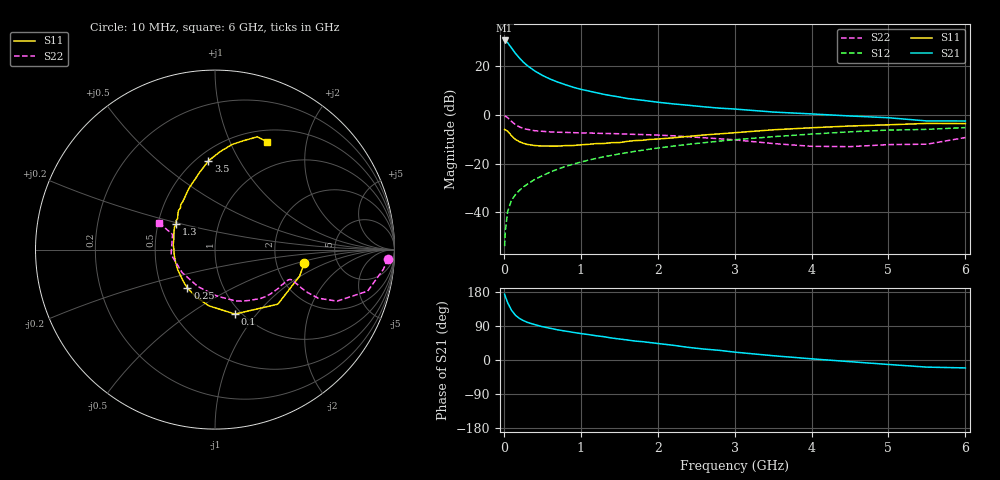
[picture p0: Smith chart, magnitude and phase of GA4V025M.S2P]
! Infineon Technologies  Discrete & RF Semiconductors
! BF775
! Si NPN RF Bipolar Junction Transistor in SOT23
! VCE = 4 V  IC = 25 mA
! Common Emitter S-Parameters:  May  1996
# GHz  S  MA  R  50
!  f  S11  S21  S12  S22
! GHz  MAG  ANG  MAG  ANG  MAG  ANG  MAG  ANG
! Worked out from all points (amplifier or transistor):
!   36 points, 10 MHz to 6 GHz, reference 50 ohm
!   highest |S21| = 30.7 dB at 10 MHz (marker M1)
!   |S21| within 3 dB of that: start of sweep to 97.65 MHz
!   unconditionally stable (mu >= 1): 338 MHz to 2.928 GHz
!   at 250 MHz: K = 0.92, MSG = 25.8 dB, |S12| = -29.7 dB
!   at 1.4 GHz: K = 1.12, MAG = 10.2 dB, |S12| = -16.6 dB
!   at 6 GHz: K = 0.94, MSG = 1.4 dB, |S12| = -5.2 dB
!   S11 on the Smith chart (normalised r, x): 10 MHz: 2.89, -0.59; 100 MHz: 0.93, -0.78; 250 MHz: 0.68, -0.31; 1.3 GHz: 0.62, +0.19; 3.5 GHz: 0.57, +0.75; 6 GHz: 0.64, +1.39
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0.01  0.5028 -8.7  34.23 173.6  0.002 87.1  0.9643 -3.1
0.02  0.4941 -17.4  33.58 167.4  0.0042 82.3  0.9452 -6.6
0.05  0.4637 -41.0  30.77 151.1  0.0104 75.2  0.8813 -15.2
0.1  0.3758 -72.8  23.95 131.3  0.0177 68.9  0.7381 -22.9
0.15  0.3151 -96.3  18.64 118.2  0.0229 66.7  0.6358 -25.2
0.2  0.2834 -111.9  15.03 110.1  0.0279 67.7  0.5719 -24.9
0.25  0.2635 -125.6  12.4 104.4  0.0327 68.1  0.5315 -24.1
0.3  0.2491 -135.8  10.55 99.8  0.0372 69.8  0.509 -23.3
0.4  0.2356 -152.1  8.115 93.5  0.0471 71.1  0.4758 -22.1
0.5  0.2301 -164.2  6.562 88.0  0.0562 71.7  0.4622 -21.5
0.6  0.2293 -172.2  5.507 83.8  0.0667 71.7  0.4498 -21.7
0.8  0.2347 173.2  4.202 76.3  0.0872 71.3  0.4393 -23.0
0.9  0.2356 167.1  3.732 73.0  0.0974 70.7  0.434 -23.7
1.1  0.2493 156.3  3.125 67.1  0.1179 69.6  0.4268 -26.4
1.3  0.2593 146.7  2.667 61.5  0.1383 67.9  0.4174 -29.1
1.6  0.2859 136.3  2.194 53.0  0.1682 64.8  0.4045 -34.7
2.2  0.339 119.3  1.695 38.9  0.2289 58.6  0.3739 -46.5
2.6  0.3876 109.6  1.475 28.9  0.2694 54.0  0.3412 -56.1
3.5  0.4961 94.2  1.151 11.3  0.3582 42.5  0.2589 -87.7
4.5  0.5938 80.7  0.955 -4.4  0.4509 28.8  0.2235 -145.0
5.5  0.6713 69.4  0.754 -18.8  0.5063 13.3  0.251 160.4
6  0.6673 64.4  0.753 -20.9  0.551 9.0  0.3441 154.5
